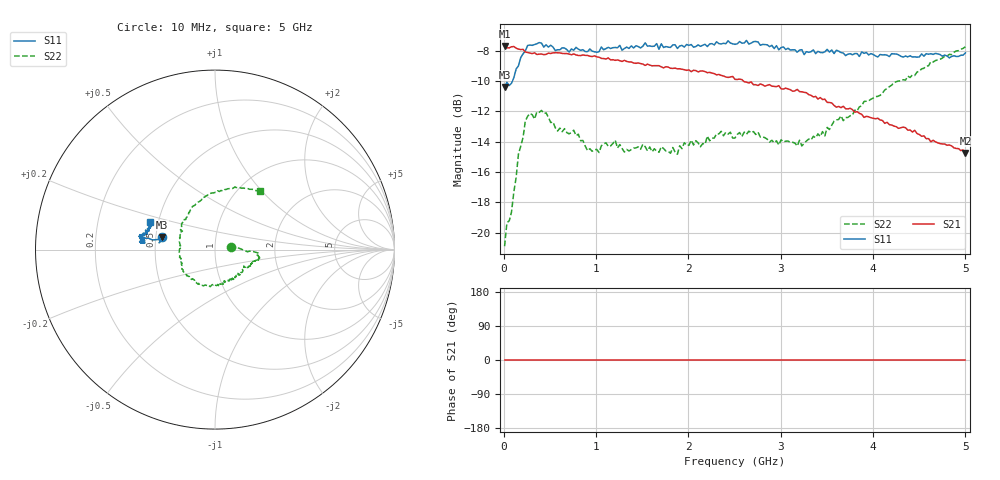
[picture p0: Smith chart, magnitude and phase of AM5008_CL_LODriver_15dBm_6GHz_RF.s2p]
!Keysight Technologies,N5245B,MY58422270,A.16.20.02
!Mixer S2P File: Scalar Mixer Measurement
!Calibration State: On
!Parameters: Stimulus Freq, S11, SC21, SC12, S22
# Hz  S  DB  R  50.0
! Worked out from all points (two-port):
!   201 points, 10 MHz to 5 GHz, reference 50 ohm
!   highest |S21| = -7.69 dB at 10 MHz (marker M1); lowest = -14.7 dB at 5 GHz (marker M2)
!   |S21| within 3 dB of the highest: start of sweep to 3.201 GHz
!   lowest |S11| = -10.4 dB at 10 MHz (marker M3), VSWR 1.87, Z = 27.1 + j4.21 ohm
!   |S11| at or under -10 dB: start of sweep to 95.04 MHz
!   |S22| runs from -20.9 to -7.7 dB; largest |S21 - S12| = 0.41
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1e7  -10.40 166.5  -7.69 0.0  -200.00 90.0  -20.89 10.8
3.495e7  -10.08 173.1  -7.81 0.0  -200.00 90.0  -19.35 3.5
8.485e7  -10.15 169.1  -7.74 0.0  -200.00 90.0  -18.64 6.9
1.597e8  -9.00 171.2  -7.90 0.0  -200.00 90.0  -14.83 -3.9
2.595e8  -7.66 170.0  -8.12 0.0  -200.00 90.0  -12.33 -4.7
4.092e8  -7.50 171.0  -8.22 0.0  -200.00 90.0  -11.94 -10.2
5.8385e8  -7.94 172.5  -8.14 0.0  -200.00 90.0  -13.30 -18.9
8.583e8  -7.94 174.0  -8.28 0.0  -200.00 90.0  -13.92 -28.7
1.03295e9  -8.07 173.7  -8.43 0.0  -200.00 90.0  -14.72 -35.6
1.2076e9  -7.79 173.6  -8.64 0.0  -200.00 90.0  -13.91 -44.8
1.3074e9  -7.86 174.3  -8.64 0.0  -200.00 90.0  -14.69 -46.0
1.68165e9  -7.91 173.3  -8.99 0.0  -200.00 90.0  -14.70 -63.2
2.13075e9  -7.72 172.1  -9.34 0.0  -200.00 90.0  -14.34 -91.7
2.2056e9  -7.73 171.6  -9.46 0.0  -200.00 90.0  -13.63 -97.3
2.505e9  -7.59 170.7  -9.89 0.0  -200.00 90.0  -13.76 -127.8
2.7545e9  -7.43 169.2  -10.30 0.0  -200.00 90.0  -13.38 -149.9
2.97905e9  -7.94 168.6  -10.31 0.0  -200.00 90.0  -14.22 -164.9
3.3533e9  -7.95 166.1  -11.05 0.0  -200.00 90.0  -13.65 161.5
3.6527e9  -8.13 164.3  -11.76 0.0  -200.00 90.0  -12.30 136.8
4.17665e9  -8.39 161.5  -12.88 0.0  -200.00 90.0  -10.37 99.7
4.62575e9  -8.20 158.9  -14.01 0.0  -200.00 90.0  -8.72 72.4
5e9  -8.15 156.9  -14.75 0.0  -200.00 90.0  -7.74 52.2
